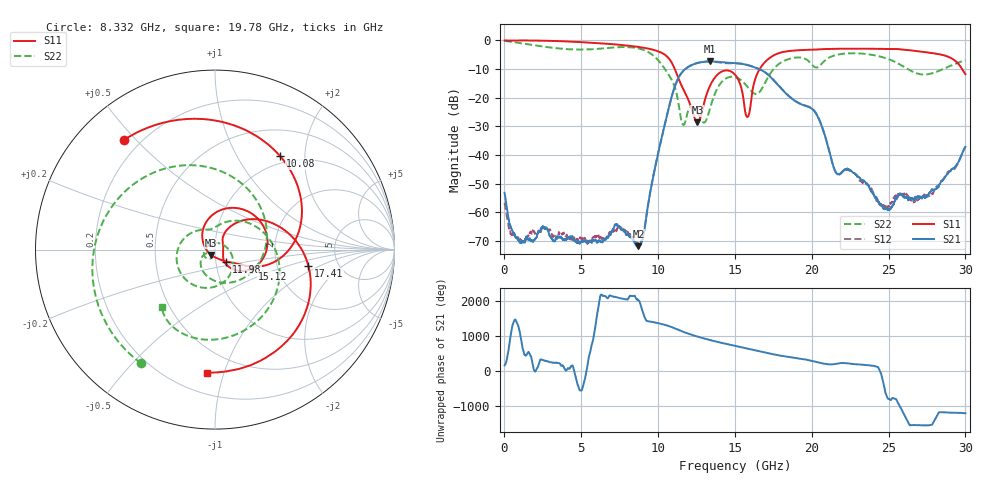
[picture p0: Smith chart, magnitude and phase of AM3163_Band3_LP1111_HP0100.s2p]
!Agilent Technologies,E8364B,MY43040894,A.07.50.67
!Agilent E8364B: A.07.50.67
!Date: Thursday, August 20, 2020 12:16:08
!Correction: S11(Full 2 Port(1,2))
!S21(Full 2 Port(1,2))
!S12(Full 2 Port(1,2))
!S22(Full 2 Port(1,2))
!S2P File: Measurements: S11, S21, S12, S22:
# Hz S  dB  R 50
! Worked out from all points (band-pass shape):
!   3201 points, 10 MHz to 30 GHz, reference 50 ohm
!   highest |S21| = -7.34 dB at 13.39 GHz (marker M1); lowest = -71.8 dB at 8.716 GHz (marker M2)
!   |S21| within 3 dB of the highest: 11.69 GHz to 16.72 GHz (5.024 GHz wide, 35.4 % of centre)
!   lowest |S11| = -28.6 dB at 12.56 GHz (marker M3), VSWR 1.08, Z = 47.7 - j2.82 ohm
!   |S11| at or under -10 dB: 11.09 GHz to 16.61 GHz (5.522 GHz wide, 39.9 % of centre); 29.78 GHz to end of sweep
!   |S22| runs from -29.5 to -0.1 dB; largest |S21 - S12| = 0.013
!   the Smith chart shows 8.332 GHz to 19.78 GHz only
!   S11 on the Smith chart (normalised r, x): 8.332 GHz: 0.14, +0.46; 10.08 GHz: 0.88, +1.53; 11.98 GHz: 1.12, -0.15; 15.12 GHz: 1.47, -0.33; 17.41 GHz: 3.03, -0.75; 19.78 GHz: 0.34, -0.88
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1e7  0.00 -2.1  -53.19 165.1  -56.66 -155.4  -0.12 -4.8
1.247088e9  -0.01 -34.0  -70.14 -166.3  -70.24 -25.0  -1.12 -82.6
2.652869e9  -0.10 -72.2  -65.57 -60.8  -65.82 57.5  -2.22 -162.8
5.014581e9  -0.59 -134.7  -70.37 164.6  -69.44 30.3  -3.20 72.2
6.617172e9  -1.13 -177.9  -69.26 -39.2  -68.85 32.8  -2.68 -17.9
8.332225e9  -2.00 129.9  -69.25 -12.4  -69.11 -136.1  -2.44 -122.9
8.716472e9  -2.26 116.3  -71.83 -131.4  -70.90 96.1  -2.77 -149.8
1.000979e10  -3.80 59.0  -39.10 -69.5  -39.13 -69.3  -6.92 90.9
1.007539e10  -3.94 55.3  -37.52 -76.0  -37.59 -75.8  -7.32 82.4
1.197788e10  -20.82 -47.0  -9.18 -10.2  -9.20 -9.9  -24.33 -121.8
1.255894e10  -28.58 -127.6  -7.87 -91.8  -7.86 -91.5  -25.20 175.8
1.339304e10  -15.66 106.2  -7.34 166.8  -7.37 166.3  -23.49 9.7
1.5005e10  -11.92 -19.2  -7.92 3.3  -7.98 5.0  -12.78 -151.2
1.511746e10  -12.70 -27.3  -7.96 -7.5  -7.98 -5.8  -12.98 -160.7
1.582972e10  -26.69 6.6  -8.62 -76.8  -8.55 -76.1  -16.26 139.6
1.741357e10  -5.55 -9.8  -13.29 128.8  -13.18 129.6  -10.68 17.2
1.978466e10  -3.26 -93.9  -23.18 -45.0  -23.04 -44.2  -7.18 -132.5
2.000958e10  -3.22 -99.6  -23.83 -67.5  -23.67 -67.0  -8.43 -137.8
2.161217e10  -2.91 -137.4  -46.34 -148.2  -46.50 -149.8  -5.04 -160.7
2.500479e10  -2.99 144.4  -59.21 -75.6  -58.15 -45.7  -6.55 68.0
2.740399e10  -4.10 77.0  -54.91 -112.6  -54.09 -95.9  -11.91 -88.3
3e10  -11.73 -28.1  -37.16 -126.6  -37.20 -127.1  -6.94 130.7
